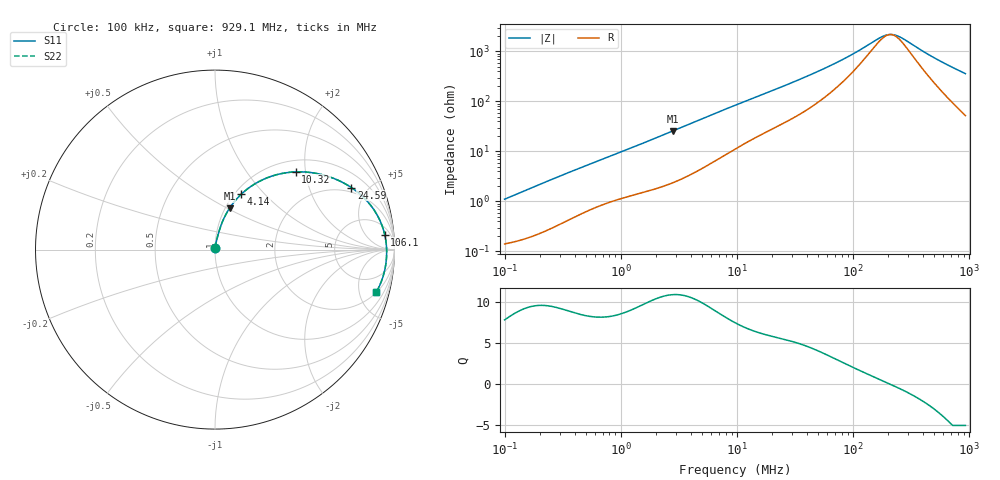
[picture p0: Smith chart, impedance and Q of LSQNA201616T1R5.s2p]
! LSQNA201616T1R5  S-PARAMETER MODEL  ( General Type )
! Model Generated by TAIYO YUDEN Corporation (http://www.ty-top.com)
! Version 2.0
! TAIYO YUDEN Control No. 100810NF25SB-FKC
! Copyright(c) 2007 TAIYO YUDEN CO.,LTD. All Rights Reserved.
! Product Description (link to TY-COMPAS)
! https://ds.yuden.co.jp/TYCOMPAS/or/detail?pn=LSQNA201616T1R5M&u=M
! Products Name : Inductors
! Characteristics :
!  Inductance : 1.5 uH , SRF(min) : 80 MHz , DC Resistance(max) : 0.143 Ohm
!  Rated Current : Saturation :550 mA , Temp Rise : 1000 mA (40 degC)
!  Case Size : 2.0 x 1.6 / 0.079 x 0.063 [mm/inch] , Thickness : 1.6 / 0.063 [mm/inch]
!  (Conditions: Temperature = 25 degC , DC Bias Current/Voltage = 0A / 0V)
! External Node Assignments :
!  1  o---GGG---o  2
! GND o---------o GND
! Frequency Range : 0.1MHz  -  929.055398MHz  [ 402 STEP ]
# MHz S RI R 50
! Freq[MHz].  S11 Real  S11 Imag  S21 Real  S21 Imag  S12 Real  S12 Imag  S22 Real  S22 Imag
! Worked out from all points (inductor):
!   401 points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, 100 kHz to 929.1 MHz, reference 50 ohm
!   read as one part in series: L = 1.75 uH near 104.7 kHz
!   highest Q = 10.8 at 2.808 MHz (marker M1), where L = 1.45 uH
!   self-resonance near 209 MHz
!   S11 on the Smith chart (normalised r, x): 100 kHz: 1.00, +0.02; 4.14 MHz: 1.07, +0.75; 10.32 MHz: 1.24, +1.77; 24.59 MHz: 1.71, +3.90; 106.1 MHz: 10, +17; 929.1 MHz: 2.04, -7.13
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0.1  0.00153 0.011  0.9985 -0.011  0.9985 -0.011  0.00153 0.011
0.462005  0.00793 0.0473  0.9921 -0.0473  0.9921 -0.0473  0.00793 0.0473
1.075699  0.022 0.0997  0.978 -0.0997  0.978 -0.0997  0.022 0.0997
2.134489  0.0538 0.1828  0.9462 -0.1828  0.9462 -0.1828  0.0538 0.1828
2.8076  0.0808 0.2303  0.9192 -0.2303  0.9192 -0.2303  0.0808 0.2303
4.139777  0.1456 0.308  0.8544 -0.308  0.8544 -0.308  0.1456 0.308
6.104059  0.2516 0.3826  0.7484 -0.3826  0.7484 -0.3826  0.2516 0.3826
9.638752  0.4222 0.4312  0.5778 -0.4312  0.5778 -0.4312  0.4222 0.4312
10.32241  0.4498 0.433  0.5502 -0.433  0.5502 -0.433  0.4498 0.433
15.22029  0.6024 0.416  0.3976 -0.416  0.3976 -0.416  0.6024 0.416
24.58924  0.7594 0.3459  0.2406 -0.3459  0.2406 -0.3459  0.7594 0.3459
33.09074  0.8307 0.2878  0.1693 -0.2878  0.1693 -0.2878  0.8307 0.2878
44.53155  0.8814 0.2278  0.1186 -0.2278  0.1186 -0.2278  0.8814 0.2278
70.31854  0.9268 0.1441  0.0732 -0.1441  0.0732 -0.1441  0.9268 0.1441
106.0796  0.9459 0.0825  0.0541 -0.0825  0.0541 -0.0825  0.9459 0.0825
171.3775  0.9549 0.0229  0.0451 -0.0229  0.0451 -0.0229  0.9549 0.0229
205.7381  0.9562 0.00179  0.0438 -0.00179  0.0438 -0.00179  0.9562 0.00179
230.6297  0.9565 -0.0114  0.0435 0.0114  0.0435 0.0114  0.9565 -0.0114
258.5329  0.9564 -0.0249  0.0436 0.0249  0.0436 0.0249  0.9564 -0.0249
513.0018  0.9445 -0.1194  0.0555 0.1194  0.0555 0.1194  0.9445 -0.1194
722.6375  0.9248 -0.1825  0.0752 0.1825  0.0752 0.1825  0.9248 -0.1825
929.0554  0.8988 -0.2373  0.1012 0.2373  0.1012 0.2373  0.8988 -0.2373
